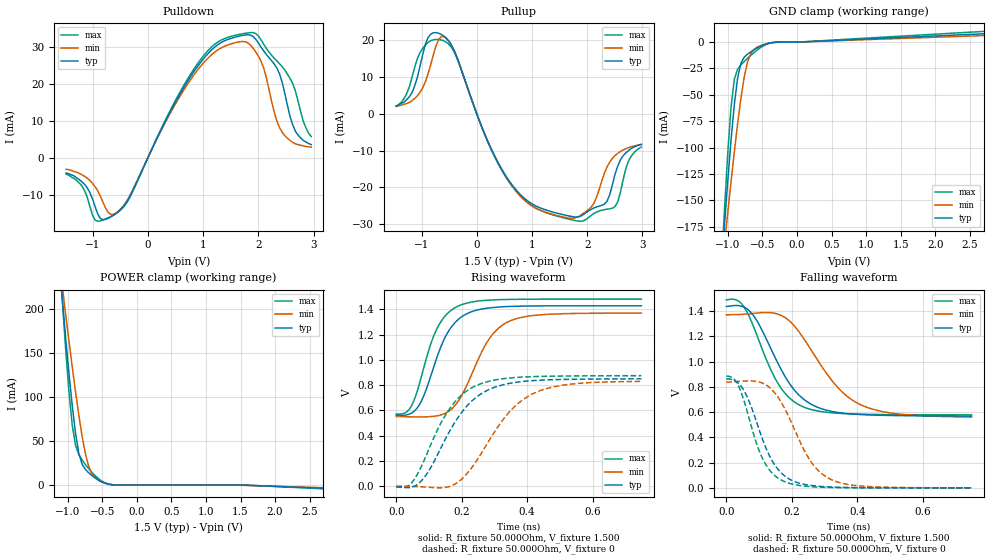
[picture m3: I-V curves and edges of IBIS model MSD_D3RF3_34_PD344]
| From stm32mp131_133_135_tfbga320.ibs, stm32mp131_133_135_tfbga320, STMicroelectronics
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[Model] MSD_D3RF3_34_PD344
Model_type   I/O
C_comp 2.325pF   2.244pF   2.446pF
Vinh = 925.000mV
Vinl = 575.000mV
Vmeas = 750.000mV
Vref = 750.000mV
[Model Spec]
Vinh   925.000mV   888.000mV   963.000mV
Vinl   575.000mV   538.000mV   613.000mV
Vmeas   750.000mV   713.000mV   788.000mV
Vref   750.000mV   713.000mV   788.000mV
[Temperature Range]   25.000   125.000   -40.000
[Voltage Range]   1.500V   1.425V   1.575V
[GND Clamp Reference]   0.00V   0.00V   0.00V
[Pulldown Reference]   0.00V   0.00V   0.00V
[POWER Clamp Reference]   1.500V   1.425V   1.575V
[Pullup Reference]   1.500V   1.425V   1.575V
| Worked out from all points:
|   slope of the pulldown table from 0 to 0.225 V, typ, clamps not added: 31.5 ohm
|   slope of the pullup table from 0 to 0.225 V, typ, clamps not added: 26.9 ohm
|   GND clamp passes 1 mA (typ) near -0.40 V on its own axis
|   POWER clamp passes 1 mA (typ) near -0.41 V on its own axis
|   rising waveform, R_fixture 50.000Ohm, V_fixture 1.500: 20-80 % time 80ps typ, 96.2ps min, 71.5ps max; typ from 0.56 V to 1.43 V
|   rising waveform, R_fixture 50.000Ohm, V_fixture 0: 20-80 % time 124ps typ, 140ps min, 111ps max; typ from -0.005 V to 0.85 V
|   falling waveform, R_fixture 50.000Ohm, V_fixture 1.500: 20-80 % time 113ps typ, 141ps min, 97.3ps max; typ from 1.44 V to 0.568 V
|   falling waveform, R_fixture 50.000Ohm, V_fixture 0: 20-80 % time 81.6ps typ, 101ps min, 70.6ps max; typ from 0.863 V to 0 V
[GND Clamp]
-1.48V    -593.9mA   -479.7mA   -763.2mA
-1.098V   -218.2mA   -223.4mA   -220.2mA
-1.05V    -174.1mA   -192.4mA   -159.6mA
-1.002V   -131.9mA   -161.9mA   -105.2mA
-954.6mV  -92.83mA   -132.3mA   -61.52mA
-906.8mV  -59.01mA   -103.9mA   -35.14mA
-859.1mV  -33.8mA    -77.16mA   -25.62mA
-811.4mV  -19.9mA    -53.08mA   -21.6mA
-715.9mV  -11.4mA    -18.73mA   -15.4mA
-572.7mV  -5.412mA   -4.636mA   -7.313mA
-334.1mV  -240.8uA   -308.8uA   -242.5uA
2.959V    8.682mA    6.832mA    11.15mA
[Power Clamp]
-1.459V   577.4mA    478.9mA    722.8mA
-1.077V   210.9mA    225.3mA    210.2mA
-1.03V    168.1mA    194.5mA    155.5mA
-981.8mV  127.5mA    164.2mA    106.7mA
-934.1mV  90.43mA    134.6mA    68.21mA
-886.4mV  58.96mA    106.1mA    45.13mA
-838.6mV  36.12mA    79.33mA    34.57mA
-743.2mV  17.82mA    35.48mA    23.27mA
-647.7mV  10.71mA    12.79mA    14.31mA
-552.3mV  5.453mA    5.392mA    7.2mA
-313.6mV  90.62uA    219.4uA    108.4uA
2.98V     -4.416mA   -3.704mA   -5.362mA
[Pulldown]
-1.48V    -4.1mA     -3.1mA     -4.4mA
-1.193V   -6.5mA     -4.6mA     -7.6mA
-954.6mV  -13.22mA   -7.8mA     -16.87mA
-811.4mV  -16.78mA   -12.04mA   -16.85mA
-572.7mV  -15.06mA   -14.91mA   -15.03mA
-334.1mV  -10.72mA   -10.48mA   -10.95mA
906.8mV   24.93mA    23.93mA    25.67mA
1.766V    33.35mA    31.48mA    33.79mA
2.052V    30.01mA    26.15mA    31.97mA
2.434V    20.42mA    6.9mA      24.74mA
2.673V    7.2mA      3.8mA      18.1mA
2.959V    3.6mA      2.9mA      5.8mA
[Pullup]
-1.459V   2.1mA      2.057mA    2.171mA
-1.173V   5.8mA      3.586mA    9.957mA
-886.4mV  20.66mA    10.7mA     19.45mA
-600mV    21.23mA    21.13mA    19.93mA
-409.1mV  17.29mA    17.18mA    16.91mA
593.2mV   -18.4mA    -18.64mA   -18.71mA
1.643V    -27.73mA   -28.34mA   -28.59mA
2.073V    -26mA      -25.39mA   -27.65mA
2.311V    -24.58mA   -16.14mA   -26.08mA
2.502V    -16.5mA    -11.36mA   -25.27mA
2.741V    -10.1mA    -9.229mA   -13.07mA
2.98V     -8.3mA     -8.343mA   -9.029mA
[Ramp]
R_load=50.000Ohm
dV/dt_r   513.720mV/102.500ps  494.399mV/119.500ps  533.820mV/91.000ps
dV/dt_f   513.720mV/97.000ps  494.399mV/122.000ps  533.820mV/84.500ps
[Rising waveform]
R_fixture=50.000Ohm
V_fixture=1.500
V_fixture_min=1.425
V_fixture_max=1.575
0s        560.4mV    551.7mV    571.8mV
39ps      569.6mV    549.5mV    605.5mV
69ps      637.6mV    548.7mV    793.3mV
123ps     1.01V      556.8mV    1.24V
154ps     1.202V     582.7mV    1.362V
192ps     1.326V     683.1mV    1.43V
276ps     1.41V      1.135V     1.473V
345ps     1.424V     1.306V     1.48V
452ps     1.429V     1.36V      1.482V
749ps     1.429V     1.371V     1.482V
[Rising waveform]
R_fixture=50.000Ohm
V_fixture=0
0s        -4.77mV    839.3uV    -4.847mV
39ps      -11.61mV   -785.7uV   5.749mV
77ps      42.12mV    -4.952mV   157.1mV
154ps     392.2mV    -8.684mV   578.9mV
199ps     581.3mV    53.5mV     720.1mV
238ps     690.4mV    172.2mV    789.1mV
330ps     805.4mV    538.9mV    852.3mV
414ps     835.6mV    728.5mV    867.5mV
529ps     846.4mV    807.1mV    873.1mV
749ps     850.5mV    830mV      875.5mV
[Falling waveform]
R_fixture=50.000Ohm
V_fixture=1.500
V_fixture_min=1.425
V_fixture_max=1.575
0s        1.435V     1.37V      1.488V
39ps      1.442V     1.372V     1.476V
77ps      1.383V     1.379V     1.315V
154ps     1.005V     1.378V     843.5mV
192ps     829.4mV    1.323V     714mV
230ps     715.5mV    1.206V     647.4mV
330ps     601.4mV    825.3mV    592.6mV
414ps     579.7mV    653.4mV    583.1mV
521ps     572mV      586.2mV    579.3mV
749ps     568.3mV    560.7mV    578.2mV
[Falling waveform]
R_fixture=50.000Ohm
V_fixture=0
0s        862.7mV    836.3mV    884.5mV
31ps      841.4mV    841.4mV    837mV
54ps      770.2mV    845.2mV    690.8mV
92ps      524.3mV    842.5mV    353mV
115ps     354.3mV    824mV      209mV
146ps     188.3mV    757.9mV    101.4mV
177ps     96.73mV    634.7mV    50.43mV
253ps     21.04mV    228.6mV    10.52mV
322ps     6.515mV    63.83mV    2.743mV
749ps     26.92uV    251.1uV    14.4uV
